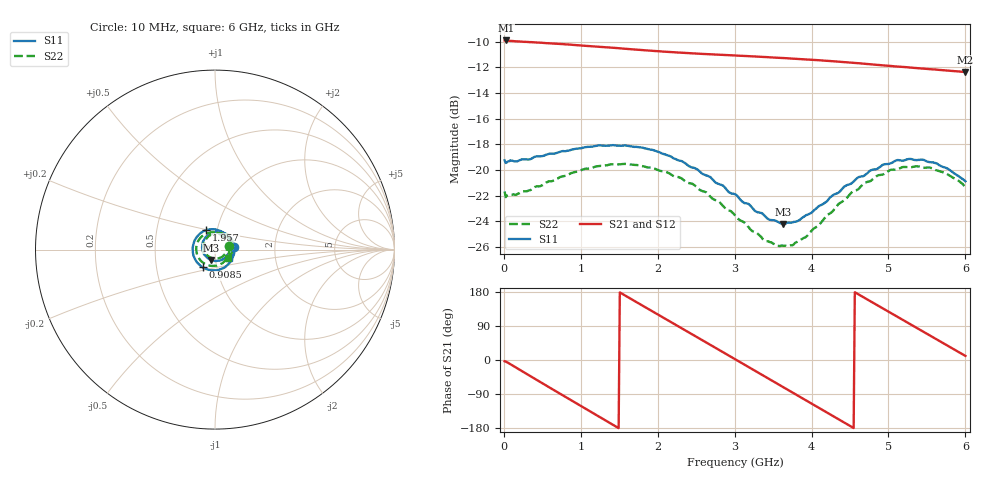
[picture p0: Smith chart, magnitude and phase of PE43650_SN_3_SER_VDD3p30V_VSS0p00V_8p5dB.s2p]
!Keysight Technologies,N5245B,MY57181451,A.13.50.07
!Date: Tuesday, May 07, 2019 08:00:01
!Correction: S11(Full 2 Port(1,2))
!S21(Full 2 Port(1,2))
!S12(Full 2 Port(1,2))
!S22(Full 2 Port(1,2))
!S2P File: Measurements: S11, S21, S12, S22:
# Hz S  dB  R 50
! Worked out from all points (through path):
!   401 points, 10 MHz to 6 GHz, reference 50 ohm
!   highest |S21| = -9.90 dB at 24.98 MHz (marker M1); lowest = -12.4 dB at 6 GHz (marker M2)
!   group delay of S21, straight-line fit = 327 ps
!   lowest |S11| = -24.2 dB at 3.634 GHz (marker M3), VSWR 1.13, Z = 47.7 - j5.56 ohm
!   |S11| at or under -10 dB: start of sweep to end of sweep
!   |S22| runs from -26.0 to -19.5 dB; largest |S21 - S12| = 0.0023
!   S11 on the Smith chart (normalised r, x): 10 MHz: 1.24, +0.04; 908.5 MHz: 0.85, -0.17; 1.957 GHz: 0.89, +0.20; 6 GHz: 1.16, -0.11
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1e7  -19.26 7.5  -9.90 -3.3  -9.93 -3.2  -21.69 13.1
2.4975e7  -19.46 0.5  -9.90 -4.2  -9.96 -4.1  -22.13 2.9
2.496e8  -19.18 -36.6  -10.00 -31.0  -10.05 -31.0  -21.68 -37.2
5.04175e8  -18.92 -72.3  -10.09 -61.8  -10.14 -61.7  -21.19 -74.1
9.085e8  -18.39 -125.2  -10.25 -110.4  -10.30 -110.4  -20.19 -126.4
1.013325e9  -18.30 -138.3  -10.30 -122.9  -10.35 -122.9  -20.00 -139.3
1.252925e9  -18.09 -166.7  -10.40 -151.4  -10.46 -151.4  -19.69 -166.9
1.47755e9  -18.11 167.2  -10.50 -178.1  -10.56 -178.1  -19.57 168.1
1.702175e9  -18.21 141.7  -10.61 155.4  -10.67 155.3  -19.61 143.8
1.95675e9  -18.48 113.6  -10.72 125.3  -10.78 125.4  -19.89 116.9
2.01665e9  -18.61 107.1  -10.74 118.3  -10.80 118.3  -20.04 110.5
2.4659e9  -19.84 56.0  -10.91 65.6  -10.97 65.6  -21.14 62.1
2.750425e9  -20.98 22.7  -11.00 32.2  -11.05 32.2  -22.36 29.2
3.005e9  -21.90 -10.9  -11.07 2.2  -11.13 2.3  -23.54 -2.5
3.289525e9  -23.28 -52.3  -11.16 -31.2  -11.21 -31.2  -24.92 -44.8
3.63395e9  -24.22 -109.4  -11.28 -71.8  -11.32 -71.8  -25.93 -103.7
4.008325e9  -23.29 -172.3  -11.41 -115.9  -11.46 -115.9  -24.70 -168.5
4.5025e9  -21.10 119.3  -11.63 -174.2  -11.68 -174.1  -21.88 122.5
4.7421e9  -20.15 90.4  -11.75 157.6  -11.80 157.8  -20.91 95.3
5.01165e9  -19.52 61.4  -11.88 126.1  -11.93 126.3  -20.05 65.5
5.4609e9  -19.22 16.6  -12.10 73.7  -12.15 73.8  -19.84 20.1
6e9  -20.89 -31.5  -12.36 10.8  -12.41 10.9  -21.33 -31.2
